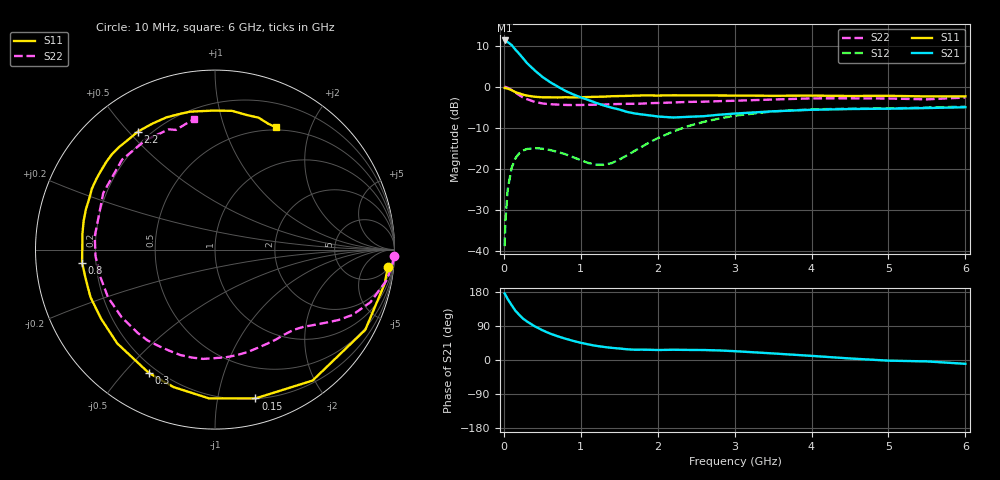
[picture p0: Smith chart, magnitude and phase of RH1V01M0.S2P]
! SIEMENS Small Signal Semiconductors
! BFR106
! Si NPN RF Bipolar Junction Transistor in SOT23
! VCE = 1 V  IC = 1 mA
! Common Emitter S-Parameters:  August  1996
# GHz  S  MA  R  50
!  f  S11  S21  S12  S22
! GHz  MAG  ANG  MAG  ANG  MAG  ANG  MAG  ANG
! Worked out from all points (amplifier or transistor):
!   36 points, 10 MHz to 6 GHz, reference 50 ohm
!   highest |S21| = 11.3 dB at 10 MHz (marker M1)
!   |S21| within 3 dB of that: start of sweep to 187.7 MHz
!   unconditionally stable (mu >= 1): 843 MHz to end of sweep
!   at 250 MHz: K = 0.30, MSG = 11.3 dB, |S12| = -15.6 dB
!   at 1.4 GHz: K = 1.58, MAG = 2.3 dB, |S12| = -18.7 dB
!   at 6 GHz: K = 1.02, MAG = -0.9 dB, |S12| = -4.9 dB
!   S11 on the Smith chart (normalised r, x): 10 MHz: 6, -18; 150 MHz: 0.20, -1.29; 300 MHz: 0.17, -0.59; 800 MHz: 0.15, -0.05; 2.2 GHz: 0.15, +0.53; 6 GHz: 0.47, +1.52
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0.01  0.9675 -5.8  3.672 175.5  0.0113 87.7  0.9986 -2.1
0.02  0.9646 -11.3  3.632 172.5  0.0225 83.0  0.9937 -4.2
0.05  0.9491 -28.1  3.512 160.9  0.0554 73.2  0.9723 -10.0
0.1  0.9099 -53.3  3.234 145.1  0.1013 59.6  0.9144 -18.7
0.15  0.8593 -74.8  2.842 130.1  0.1335 47.3  0.8482 -25.4
0.2  0.8296 -92.3  2.525 119.2  0.154 38.7  0.7904 -29.8
0.25  0.8 -106.8  2.224 109.2  0.1665 31.2  0.737 -33.6
0.3  0.7798 -118.2  1.948 101.7  0.1735 26.2  0.7043 -36.3
0.4  0.7549 -136.2  1.587 89.1  0.1783 17.8  0.6543 -41.1
0.5  0.7423 -148.7  1.321 78.7  0.1752 12.4  0.6254 -45.7
0.6  0.7427 -159.1  1.139 69.8  0.1686 8.7  0.6114 -50.7
0.8  0.7442 -174.4  0.89 56.3  0.1499 6.2  0.5993 -61.2
1.1  0.749 167.7  0.688 41.1  0.117 15.3  0.6007 -78.4
1.4  0.7654 153.7  0.555 32.1  0.1164 40.2  0.6126 -96.3
1.8  0.7822 137.3  0.458 27.3  0.1863 58.7  0.6221 -120.3
2.2  0.7853 123.1  0.421 27.0  0.2841 56.6  0.6424 -144.1
2.8  0.7813 104.9  0.455 25.2  0.4091 43.0  0.6666 -176.8
3.5  0.7747 90.4  0.501 17.3  0.5001 26.5  0.6981 153.1
4.5  0.7706 76.8  0.534 4.0  0.5397 7.8  0.7221 122.3
5  0.774 71.7  0.54 -1.7  0.5433 1.0  0.7178 111.0
5.5  0.7609 66.9  0.549 -3.7  0.5575 -2.3  0.7015 108.1
6  0.762 63.3  0.562 -10.1  0.5708 -9.1  0.738 99.0
